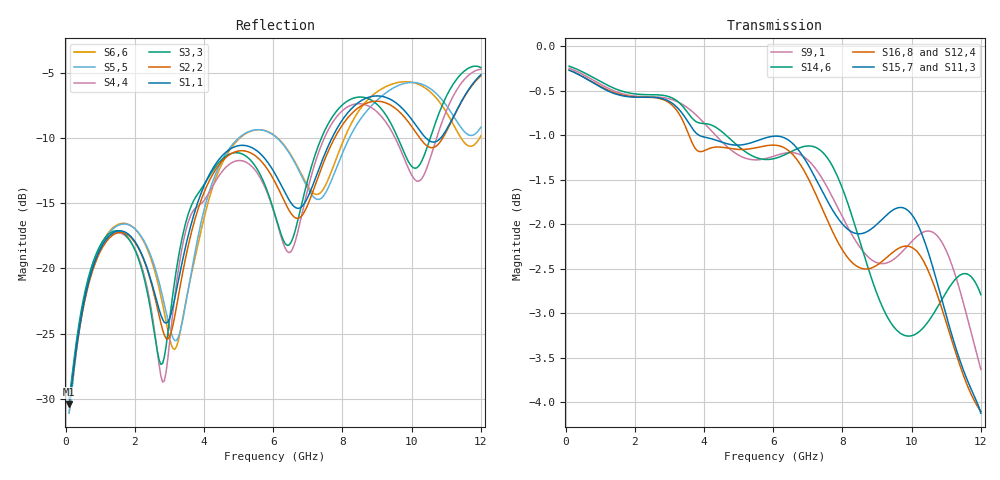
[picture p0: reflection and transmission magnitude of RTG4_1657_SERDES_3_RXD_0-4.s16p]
! RTG4 1657 S-parameter file
! Microsemi Corporation (c) 2019
!Initial ver: Jul 30, 2019
! Port::PIN_NAME::NET_NAME::S-parameter ports::PORT SIDE
! Port1:--:SERDES_3_RXD0_N_DIE::1::DIE
! Port2:--:SERDES_3_RXD0_P_DIE::2::DIE
! Port3:AY23:SERDES_3_RXD0_N_BGA::3::BGA
! Port4:BA23:SERDES_3_RXD0_P_BGA::4::BGA
! Port5:--:SERDES_3_RXD1_N_DIE::5::DIE
! Port6:--:SERDES_3_RXD1_P_DIE::6::DIE
! Port7:AY25:SERDES_3_RXD1_N_BGA::7::BGA
! Port8:BA25:SERDES_3_RXD1_P_BGA::8::BGA
! Port9:--:SERDES_3_RXD2_N_DIE::9::DIE
! Port10:--:SERDES_3_RXD2_P_DIE::10::DIE
! Port11:AV26:SERDES_3_RXD2_N_BGA::11::BGA
! Port12:AW26:SERDES_3_RXD2_P_BGA::12::BGA
! Port13:--:SERDES_3_RXD3_N_DIE::13::DIE
! Port14:--:SERDES_3_RXD3_P_DIE::14::DIE
! Port15:AY27:SERDES_3_RXD3_N_BGA::15::BGA
! Port16:BA27:SERDES_3_RXD3_P_BGA::16::BGA
!TouchstoneFormatFlag = 1
! GNDNET
! NETSLIST
! User Comments:
! Touchstone file exported from HFSS 2018.2.0
!  File:  //LSI_Z840_SIM_PC/Simulation_Data/MASUMISU/Microsemi_190710/YBD197_150320_NETCHANGE_SERDES_3_RXD.aedt
!  Generated:  8:55:33 ??  7 16, 2019
!  Design:  HFSSModel1
!  Project:  YBD197_150320_NETCHANGE_SERDES_3_RXD
!  Setup:  Setup1
!  Solution:  Sweep
! Terminal data exported
! Port[1] = SERDES_3_RXD0_N_DIE
! Port[2] = SERDES_3_RXD0_P_DIE
! Port[3] = SERDES_3_RXD1_N_DIE
! Port[4] = SERDES_3_RXD1_P_DIE
! Port[5] = SERDES_3_RXD2_N_DIE
! Port[6] = SERDES_3_RXD2_P_DIE
! Port[7] = SERDES_3_RXD3_N_DIE
! Port[8] = SERDES_3_RXD3_P_DIE
! Port[9] = SERDES_3_RXD0_N_BGA
! Port[10] = SERDES_3_RXD0_P_BGA
! Port[11] = SERDES_3_RXD1_N_BGA
! Port[12] = SERDES_3_RXD1_P_BGA
! Port[13] = SERDES_3_RXD2_N_BGA
! Port[14] = SERDES_3_RXD2_P_BGA
! Port[15] = SERDES_3_RXD3_N_BGA
! Port[16] = SERDES_3_RXD3_P_BGA
# GHZ S DB R 50.000000
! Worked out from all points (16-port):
!   239 points, 100 MHz to 12 GHz, reference 50 ohm
!   strongest paths, dB at 100 MHz, 3.05 GHz, 6.05 GHz, 9.05 GHz, 12 GHz:
!     S15,7: -0.3, -0.6, -1.0, -2.0, -4.1
!     S11,3: -0.3, -0.6, -1.0, -2.2, -5.0
!     S16,8: -0.3, -0.7, -1.1, -2.4, -4.1
!     S12,4: -0.3, -0.7, -1.1, -2.6, -4.4
!     S14,6: -0.2, -0.6, -1.3, -2.8, -2.8
!     S9,1: -0.2, -0.6, -1.2, -2.4, -3.6
!   lowest |S11| = -30.4 dB at 100 MHz (marker M1), VSWR 1.06, Z = 52.6 - j1.62 ohm
!   |S11| at or under -10 dB: start of sweep to 7.699 GHz; 10.41 GHz to 10.84 GHz (437 MHz wide, 4.11 % of centre)
